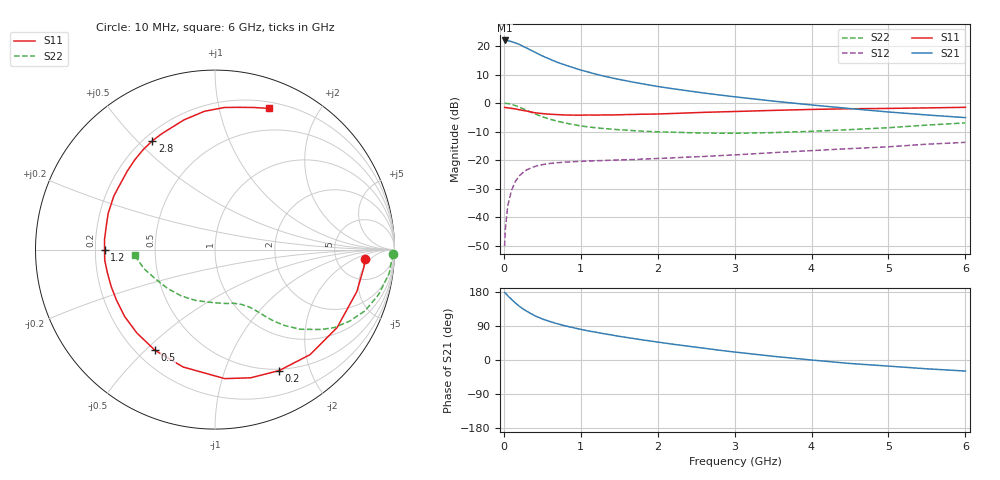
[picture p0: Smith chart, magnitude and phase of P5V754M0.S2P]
! SIEMENS Small Signal Semiconductors
! BFP183
! Si NPN RF Bipolar Junction Transistor in SOT143
! VCE = 0.75 V  IC = 4 mA
! Common Emitter S-Parameters:  March  1996
# GHz  S  MA  R  50
!  f  S11  S21  S12  S22
! GHz  MAG  ANG  MAG  ANG  MAG  ANG  MAG  ANG
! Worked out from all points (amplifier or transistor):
!   36 points, 10 MHz to 6 GHz, reference 50 ohm
!   highest |S21| = 21.9 dB at 10 MHz (marker M1)
!   |S21| within 3 dB of that: start of sweep to 321.2 MHz
!   unconditionally stable (mu >= 1): 1.595 GHz to end of sweep
!   at 250 MHz: K = 0.19, MSG = 22.1 dB, |S12| = -24.3 dB
!   at 1.4 GHz: K = 0.92, MSG = 14.4 dB, |S12| = -20.0 dB
!   at 6 GHz: K = 1.07, MAG = 2.7 dB, |S12| = -13.8 dB
!   S11 on the Smith chart (normalised r, x): 10 MHz: 10, -3; 200 MHz: 0.48, -1.56; 500 MHz: 0.27, -0.54; 1.2 GHz: 0.24, +0.00; 2.8 GHz: 0.23, +0.55; 6 GHz: 0.26, +1.42
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0.01  0.837 -3.4  12.5 178.2  0.0031 85.1  0.9935 -1.5
0.02  0.8354 -6.7  12.41 176.4  0.0062 86.6  0.9869 -3.2
0.05  0.8241 -16.5  12.42 169.7  0.0157 82.9  0.9793 -7.8
0.1  0.8073 -32.6  11.91 159.8  0.0295 72.2  0.9449 -15.4
0.15  0.7892 -47.9  11.3 150.5  0.0424 65.0  0.9029 -22.2
0.2  0.763 -62.0  10.69 142.0  0.0527 58.8  0.8492 -28.0
0.25  0.7415 -74.4  9.848 134.6  0.0608 52.8  0.7946 -33.1
0.3  0.7208 -85.7  9.145 128.5  0.0678 48.2  0.7413 -36.9
0.4  0.6778 -105.2  7.82 117.0  0.0772 40.3  0.6509 -43.0
0.5  0.653 -120.8  6.697 108.3  0.0832 35.0  0.5753 -47.4
0.6  0.6367 -133.1  5.869 101.4  0.0874 31.1  0.5202 -50.3
0.7  0.6265 -143.5  5.139 95.4  0.0899 28.2  0.4783 -52.4
0.9  0.6139 -160.4  4.179 85.4  0.0938 24.6  0.4196 -55.5
1.1  0.6172 -174.5  3.483 76.6  0.0964 22.4  0.3808 -58.3
1.2  0.6154 180.0  3.199 73.2  0.0976 21.5  0.3683 -59.8
1.7  0.6314 156.4  2.296 56.2  0.1023 20.5  0.3274 -67.4
2.2  0.6563 138.0  1.778 41.6  0.1095 20.8  0.3083 -77.0
2.8  0.6991 120.0  1.386 25.8  0.1198 21.5  0.2958 -91.6
3.5  0.743 103.5  1.081 9.8  0.1349 21.1  0.3032 -110.9
4.5  0.7936 86.2  0.8 -9.2  0.1589 18.0  0.3422 -140.9
5.5  0.8219 74.4  0.618 -23.3  0.19 13.9  0.4107 -165.1
6  0.8416 69.2  0.555 -29.1  0.2045 10.2  0.4482 -176.0
